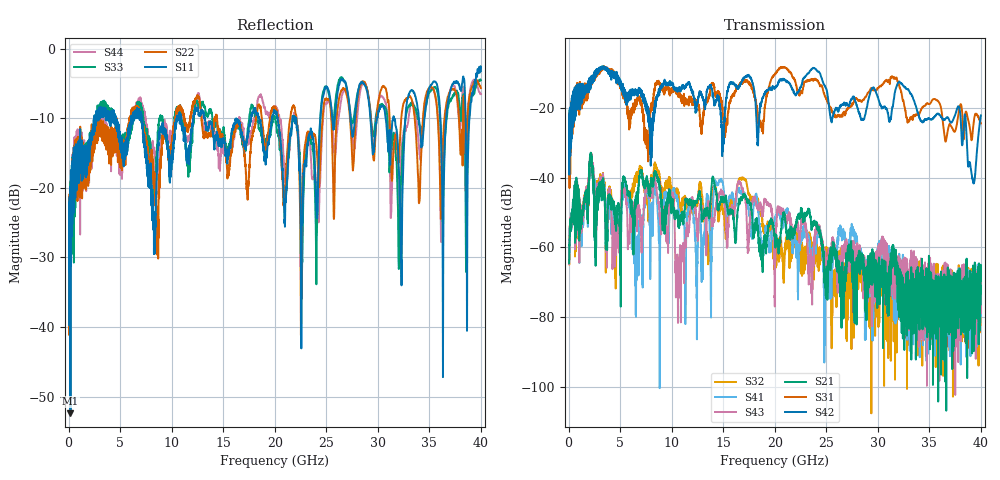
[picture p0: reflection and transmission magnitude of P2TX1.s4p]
!Agilent Technologies,N5245A,MY49151084,A.09.20.08
!Agilent N5245A: A.09.20.08
!Date: Thursday, March 01, 2012 14:41:07
!Correction: S11(Full 4 Port(1,2,3,4))
!S12(Full 4 Port(1,2,3,4))
!S13(Full 4 Port(1,2,3,4))
!S14(Full 4 Port(1,2,3,4))
!S21(Full 4 Port(1,2,3,4))
!S22(Full 4 Port(1,2,3,4))
!S23(Full 4 Port(1,2,3,4))
!S24(Full 4 Port(1,2,3,4))
!S31(Full 4 Port(1,2,3,4))
!S32(Full 4 Port(1,2,3,4))
!S33(Full 4 Port(1,2,3,4))
!S34(Full 4 Port(1,2,3,4))
!S41(Full 4 Port(1,2,3,4))
!S42(Full 4 Port(1,2,3,4))
!S43(Full 4 Port(1,2,3,4))
!S44(Full 4 Port(1,2,3,4))
!S4P File: Measurements: <S11,S12,S13,S14>,
!<S21,S22,S23,S24>,
!<S31,S32,S33,S34>,
!<S41,S42,S43,S44>:
# Hz S  dB  R 50
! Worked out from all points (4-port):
!   3996 points, 50 MHz to 40 GHz, reference 50 ohm
!   strongest paths, dB at 50 MHz, 10.04 GHz, 20.03 GHz, 30.02 GHz, 40 GHz:
!     S42: -24.9, -13.0, -14.3, -17.1, -22.1
!     S31: -27.2, -14.4, -10.1, -14.4, -24.5
!     S21: -64.5, -46.2, -57.9, -64.9, -69.6
!     S43: -64.8, -45.6, -63.0, -61.7, -78.7
!     S41: -64.3, -45.7, -52.0, -59.9, -79.6
!     S32: -62.2, -42.7, -58.7, -67.9, -66.7
!   lowest |S11| = -52.4 dB at 180 MHz (marker M1), VSWR 1.00, Z = 50.2 - j0.107 ohm
!   |S11| at or under -10 dB: start of sweep to 2.508 GHz; 7.102 GHz to 10.52 GHz (3.415 GHz wide, 38.8 % of centre); 13.22 GHz to 17.7 GHz (4.483 GHz wide, 29 % of centre)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
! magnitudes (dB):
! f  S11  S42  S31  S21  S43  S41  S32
! 50 MHz  -25.6  -24.9  -27.2  -64.5  -64.8  -64.3  -62.2
! 180 MHz  -52.4  -31.6  -29.3  -54.4  -53.8  -54.7  -53.9
! 8.36 GHz  -26.7  -18.5  -14.8  -38.1  -39.6  -41.9  -36.0
! 10.57 GHz  -9.7  -14.5  -15.8  -49.6  -63.1  -46.1  -44.2
! 16.82 GHz  -12.4  -12.5  -12.8  -46.5  -43.3  -44.3  -40.5
! 25.61 GHz  -10.4  -22.6  -21.4  -62.3  -59.1  -63.2  -70.3
! 40 GHz  -3.2  -22.1  -24.5  -69.6  -78.7  -79.6  -66.7
